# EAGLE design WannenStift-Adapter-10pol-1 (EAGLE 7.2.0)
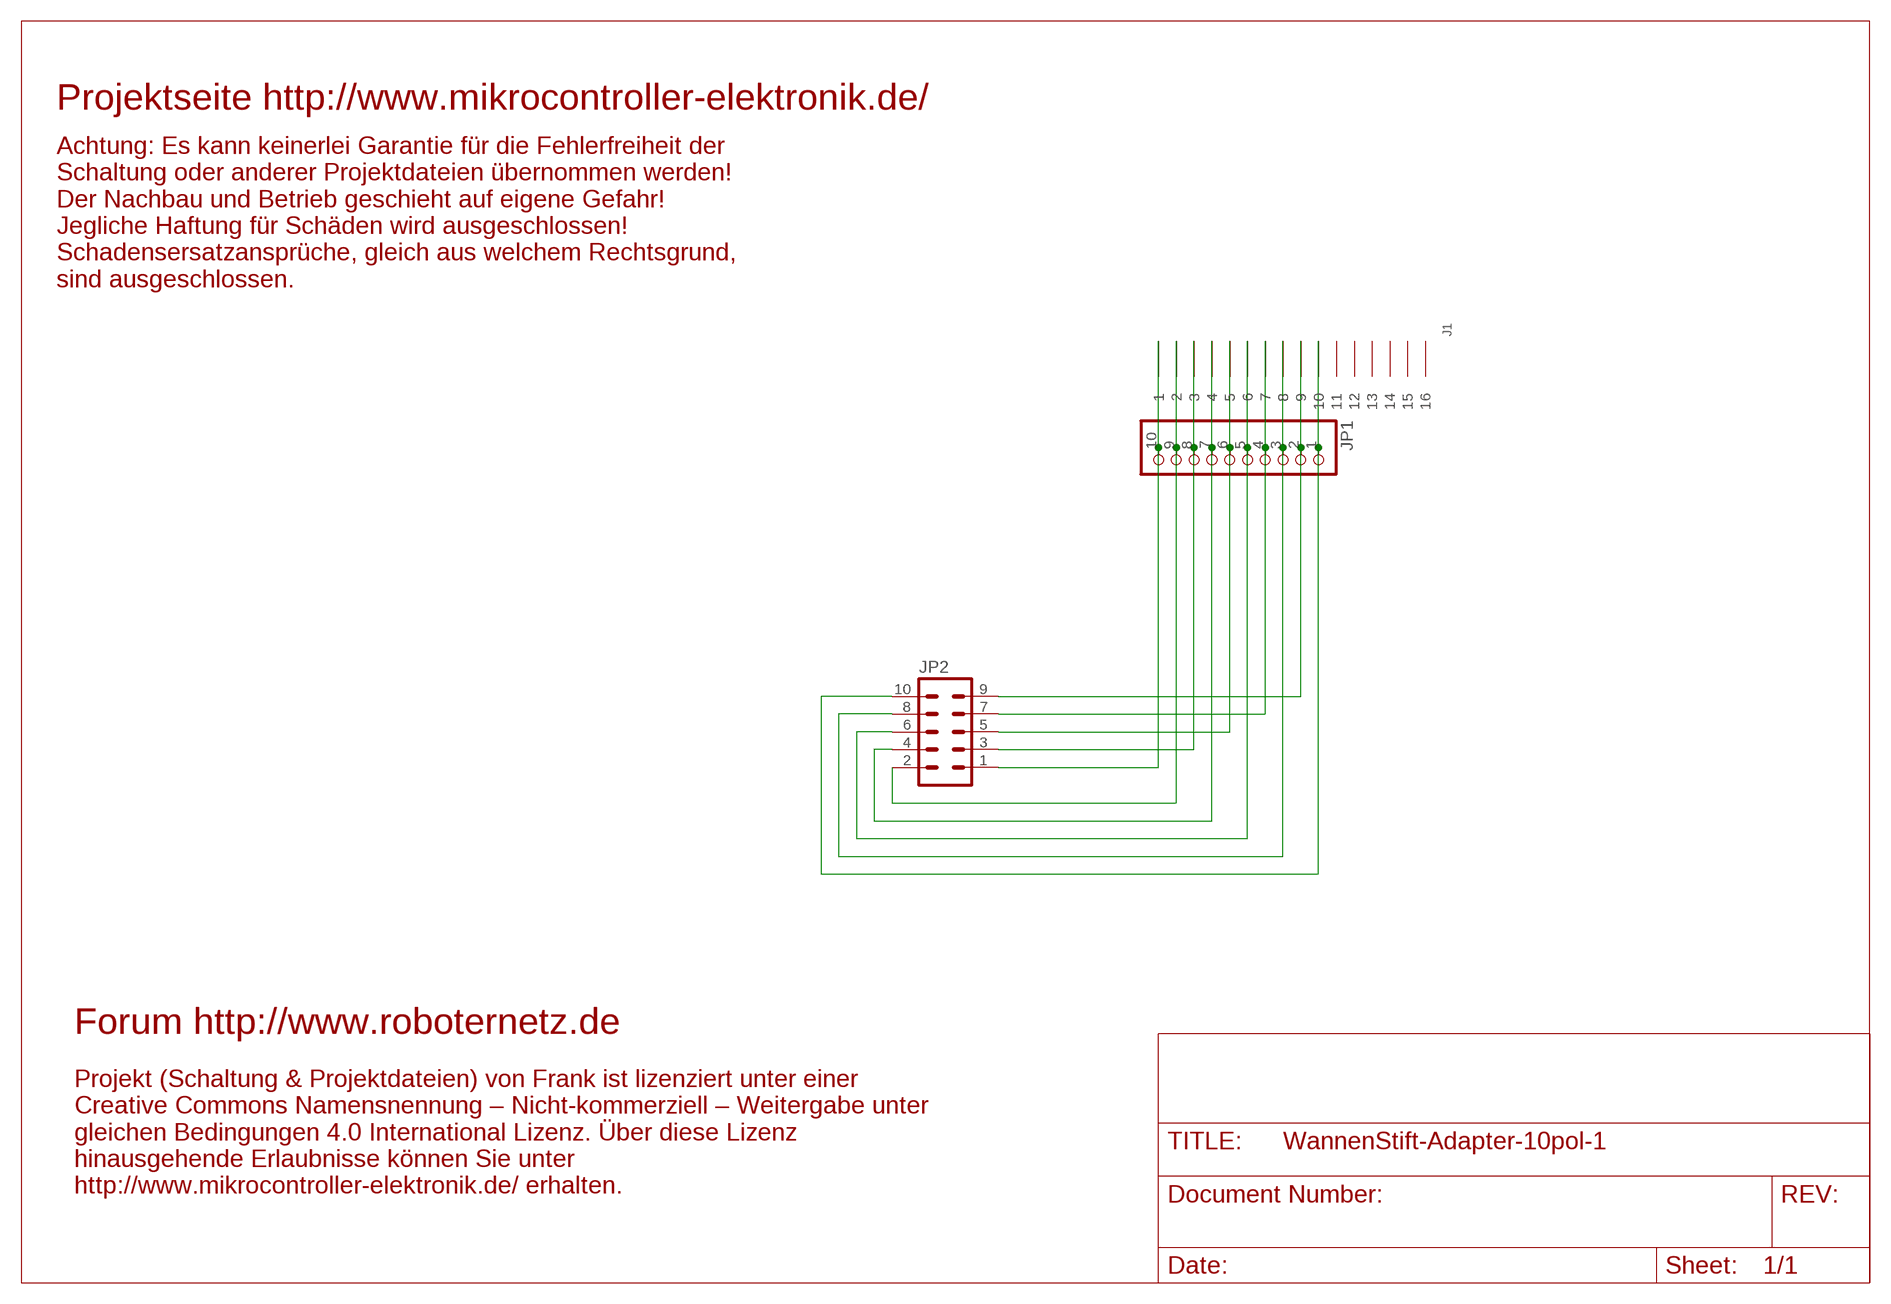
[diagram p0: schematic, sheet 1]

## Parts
J1  LOETFLAECHE-SMD-2X8LOETFLAECHE-2X8  [LOETFLAECHE-SMD-2X8]
JP1  PINHD-1X10  [1X10]
JP2  ML10  [ML10]

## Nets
JP1: J1.1 JP1.10 JP2.1
N$1: J1.5 JP1.6 JP2.5
N$2: J1.2 JP1.9 JP2.2
N$3: J1.3 JP1.8 JP2.3
N$4: J1.4 JP1.7 JP2.4
N$5: J1.6 JP1.5 JP2.6
N$6: J1.7 JP1.4 JP2.7
N$7: J1.8 JP1.3 JP2.8
N$8: J1.9 JP1.2 JP2.9
N$9: J1.10 JP1.1 JP2.10
Unconnected: J1.11 J1.12 J1.13 J1.14 J1.15 J1.16

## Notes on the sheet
- Projektseite http://www.mikrocontroller-elektronik.de/
- Achtung: Es kann keinerlei Garantie für die Fehlerfreiheit der
  Schaltung oder anderer Projektdateien übernommen werden!
  Der Nachbau und Betrieb geschieht auf eigene Gefahr! 
  Jegliche Haftung für Schäden wird ausgeschlossen!
  Schadensersatzansprüche, gleich aus welchem Rechtsgrund,
  sind ausgeschlossen.
- Forum http://www.roboternetz.de
- Projekt (Schaltung & Projektdateien) von Frank ist lizenziert unter einer
  Creative Commons Namensnennung – Nicht-kommerziell – Weitergabe unter
  gleichen Bedingungen 4.0 International Lizenz. Über diese Lizenz
  hinausgehende Erlaubnisse können Sie unter
  http://www.mikrocontroller-elektronik.de/ erhalten.

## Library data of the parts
J1 = RoboterNetzNeu:LOETFLAECHE-SMD-2X8: LOETFLAECHE-SMD-2X8
JP1 = pinhead:PINHD-1X10: PIN HEADER
JP2 = con-ml:ML10: HARTING; OC_FARNELL: unknown; OC_NEWARK: unknown

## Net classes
0 default: width 0.254 mm

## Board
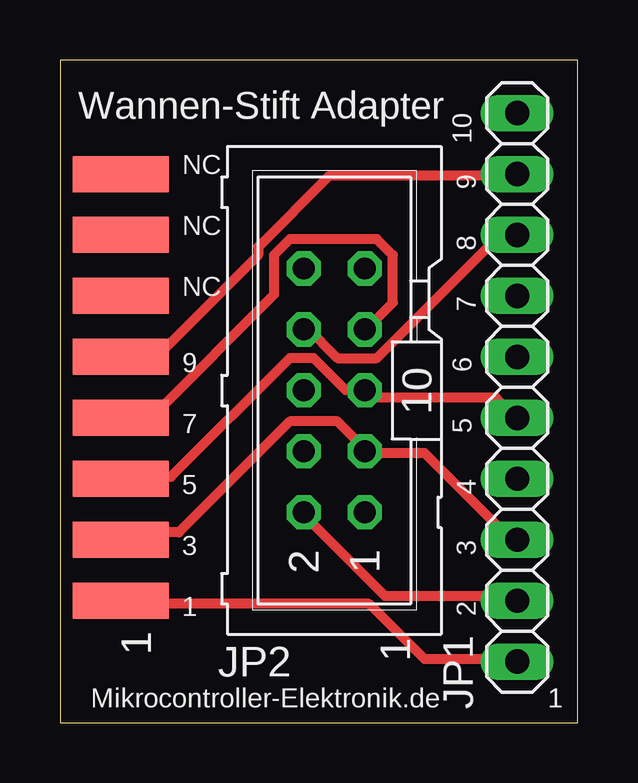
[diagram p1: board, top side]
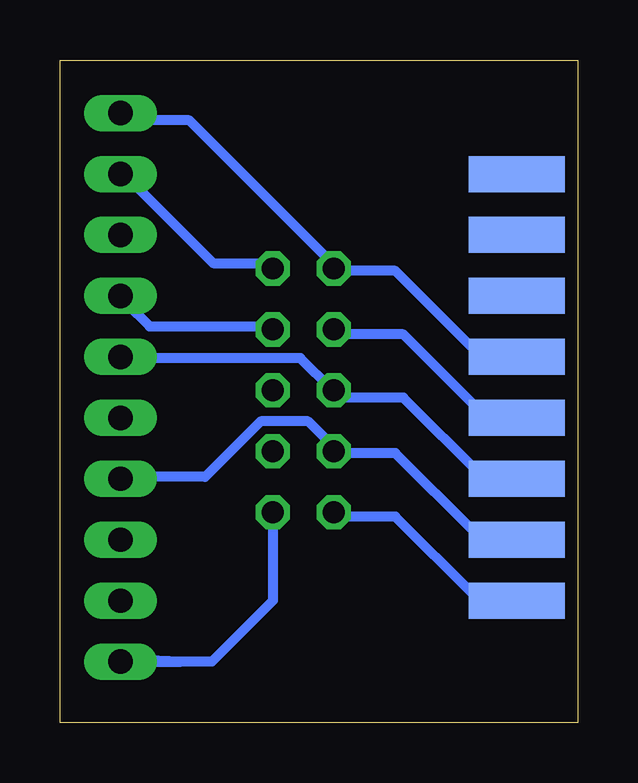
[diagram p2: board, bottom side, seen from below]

Size 21.57 x 27.61 mm. Coordinates in mm from the lower left corner, seen from the top.
Outline: 0,0 21.57,0 21.57,27.61 0,27.61 0,0
Copper layers (1*16): Top 0.035mm / dielectric 1.5mm / Bottom 0.035mm
Design rules "default *": minimum track width 16mil, minimum drill 24mil, track to track 10mil, track to pad 10mil, pad to pad 12mil, via to via 12mil, smd to smd 12mil, copper to edge 40mil, drill to drill 8mil, minimum pad ring 10mil, minimum via ring 8mil, stop-mask expansion 4mil, vias tented up to drill 0mil, thermal gap 10mil

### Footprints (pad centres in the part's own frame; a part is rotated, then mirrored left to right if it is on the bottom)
LOETFLAECHE-SMD-2X8 = smd 4 x 1.5: 1 0,-7.62; 3 0,-5.08; 5 0,-2.54; 7 0,0; 9 0,2.54; 11 0,5.08; 13 0,7.62; 15 0,10.16 | smd 4 x 1.5 bottom: 2 0,-7.62; 4 0,-5.08; 6 0,-2.54; 8 0,0; 10 0,2.54; 12 0,5.08; 14 0,7.62; 16 0,10.16
1X10 = drill 1.016 long: 1 -11.43,0; 2 -8.89,0; 3 -6.35,0; 4 -3.81,0; 5 -1.27,0; 6 1.27,0; 7 3.81,0; 8 6.35,0; 9 8.89,0; 10 11.43,0
ML10 = drill 0.914 octagon: 1 -5.08,-1.27; 2 -5.08,1.27; 3 -2.54,-1.27; 4 -2.54,1.27; 5 0,-1.27; 6 0,1.27; 7 2.54,-1.27; 8 2.54,1.27; 9 5.08,-1.27; 10 5.08,1.27

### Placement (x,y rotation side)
J1  2.54,12.7 0 top
JP1  19.05,13.97 270 top
JP2  11.43,13.84 90 top

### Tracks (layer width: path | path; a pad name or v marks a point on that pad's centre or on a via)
JP1
  Top 0.406: J1.1 2.64,4.95 12.88,4.95 15.19,2.64 18.82,2.64 JP1.10
  Bottom 0.406: JP2.1 12.7,5.08 15.24,2.54 16.51,2.54 | 17.78,2.54 16.51,2.54 | 16.51,2.54 18.82,2.64 JP1.10
N$1
  Top 0.406: JP1.6 18.82,12.88 18.16,13.54 12.88,13.54 JP2.5 12.55,13.87 11.89,13.87 10.57,15.19 9.58,15.19 4.62,10.24 2.64,10.24 J1.5
N$2
  Top 0.406: JP1.9 18.82,5.28 13.54,5.28 10.24,8.59 JP2.2
  Bottom 0.406: JP2.2 9.91,8.59 7.59,8.59 4.29,5.28 2.64,5.28 J1.2
N$3
  Top 0.406: JP1.8 18.82,7.59 15.19,11.23 12.88,11.23 JP2.3 12.55,11.56 11.56,12.55 9.58,12.55 4.95,7.92 2.64,7.92 J1.3
N$4
  Bottom 0.406: J1.4 2.64,7.92 4.29,7.92 7.59,11.23 9.91,11.23 JP2.4 10.24,11.56 11.23,12.55 13.21,12.55 15.52,10.24 18.82,10.24 JP1.7
N$5
  Bottom 0.406: J1.6 2.64,10.24 3.96,10.24 7.26,13.54 9.91,13.54 JP2.6 10.24,13.87 11.56,15.19 18.82,15.19 JP1.5
N$6
  Top 0.406: J1.7 2.64,12.88 3.96,12.88 8.91,17.83 8.91,19.48 9.58,20.14 13.21,20.14 13.87,19.48 13.87,17.5 12.88,16.51 JP2.7
  Bottom 0.406: JP2.7 12.88,16.51 17.83,16.51 18.82,17.5 JP1.4
N$7
  Top 0.406: JP1.3 18.82,20.14 18.16,20.14 13.21,15.19 11.56,15.19 10.24,16.51 JP2.8
  Bottom 0.406: JP2.8 9.91,16.18 7.26,16.18 3.96,12.88 2.64,12.88 J1.8
N$8
  Top 0.406: J1.9 2.64,15.52 4.29,15.52 8.26,19.48 8.26,19.81 11.23,22.78 18.82,22.78 JP1.2
  Bottom 0.406: JP2.9 12.88,19.15 15.19,19.15 18.82,22.78 JP1.2
N$9
  Bottom 0.406: J1.10 2.64,15.52 4.29,15.52 7.59,18.82 9.91,18.82 JP2.10 10.24,19.15 16.18,25.09 18.82,25.09 JP1.1

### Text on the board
tPlace: Wannen-Stift Adapter | 10 | NC | 9 | NC | 8 | NC | 7 | 9 | 6 | 7 | 5 | 5 | 4 | 3 | 3 | 2 | 1 | 1 | Mikrocontroller-Elektronik.de | 1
